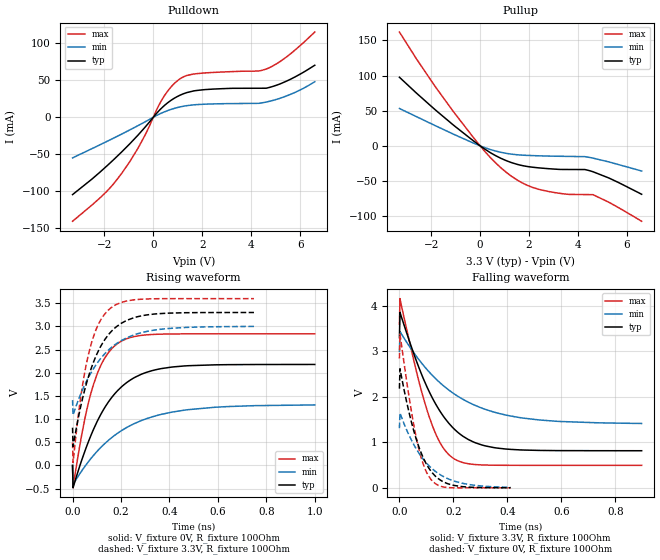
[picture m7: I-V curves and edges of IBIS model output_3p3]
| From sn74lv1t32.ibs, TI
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|   output_3p3 Model
[Model]   output_3p3
Model_type   Output
Polarity   Inverting
Vmeas = 1.65
Vref = 0
Cref = 30pF
Rref = 150
|   typ   min   max
|   (nom PVT)   (fast PVT)   (slow PVT)
C_comp   1.702e-12   1.593e-12   1.765e-12
| Where nom  PVT is Nominal Process, 3.3V, 40C
|   Fast PVT is Strong Process,  3.6V, -40C
|   Slow PVT is Weak Process,   3V, 140C
[Voltage Range]   3.3   3   3.6
|Junction Temperature
[Temperature Range]   40   140   -40
[Pullup Reference]   3.3   3   3.6
[Pulldown Reference]   0   0   0
[Power Clamp Reference]   3.3   3   3.6
[GND Clamp Reference]   0   0   0
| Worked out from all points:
|   slope of the pulldown table from 0 to 0.495 V, typ, clamps not added: 29 ohm
|   slope of the pullup table from 0 to 0.495 V, typ, clamps not added: 43.9 ohm
|   falling waveform, V_fixture 3.3V, R_fixture 100Ohm: 20-80 % time 138ps typ, 225ps min, 93.8ps max; typ from 3.3 V to 0.815 V
|   rising waveform, V_fixture 0V, R_fixture 100Ohm: 20-80 % time 153ps typ, 232ps min, 93.4ps max; typ from 0 V to 2.18 V
|   rising waveform, V_fixture 3.3V, R_fixture 100Ohm: 20-80 % time 110ps typ, 148ps min, 76.2ps max; typ from 0.815 V to 3.3 V
|   falling waveform, V_fixture 0V, R_fixture 100Ohm: 20-80 % time 76.3ps typ, 112ps min, 57ps max; typ from 2.18 V to 0.002 V
[Pulldown]
|   Voltage   I(typ)   I(min)   I(max)
-3.3V     -104.5mA   -54.85mA   -140.5mA
-1.896V   -65.69mA   -32.59mA   -99.89mA
-1.291V   -46.79mA   -22.65mA   -75.76mA
-618mV    -23.85mA   -11.17mA   -41.41mA
408mV     14.56mA    6.683mA    26.68mA
746.4mV   23.38mA    10.87mA    41.78mA
1.049V    29.16mA    13.66mA    51mA
1.373V    33.38mA    15.72mA    56.48mA
2.043V    37.19mA    17.6mA     59.75mA
4.609V    39.26mA    20.53mA    65.09mA
5.448V    48.87mA    28.84mA    81.62mA
6.6V      70.29mA    47.98mA    115.2mA
[Pullup]
|   Voltage   I(typ)   I(min)   I(max)
-3.3V     97.54mA    53.13mA    161.8mA
-1.882V   52.63mA    29.49mA    86.56mA
-1.043V   28.1mA     15.84mA    46.36mA
194.7mV   -4.752mA   -2.606mA   -8.053mA
1.079V    -21.23mA   -10.73mA   -37.97mA
1.736V    -28.14mA   -13.22mA   -52.95mA
2.376V    -31.23mA   -14.13mA   -61.59mA
3.627V    -33.6mA    -15mA      -69.02mA
4.446V    -35.06mA   -16.32mA   -69.31mA
4.61V     -36.79mA   -17.43mA   -69.37mA
5.25V     -45.55mA   -22.74mA   -80.01mA
6.6V      -68.82mA   -35.76mA   -107.2mA
[Ramp]
R_load = 100
|   typ   min   max
dV/dt_r   1.30758/1.52632e-10   0.783735/2.32218e-10   1.70409/9.33057e-11
dV/dt_f   1.49085/1.37591e-10   0.951762/2.2497e-10   1.8634/9.37035e-11
[Falling Waveform]
V_fixture = 3.3V
V_fixture_min = 3V
V_fixture_max = 3.6V
R_fixture = 100Ohm
|   Time   V(typ)   V(min)   V(max)
0s        3.3V       3V         3.6V
2ps       3.858V     3.435V     4.159V
68ps      2.708V     2.849V     2.437V
112ps     2.093V     2.535V     1.535V
152ps     1.669V     2.301V     976.8mV
202ps     1.298V     2.068V     640.4mV
276ps     1.003V     1.824V     514.1mV
366ps     870.9mV    1.64V      496.1mV
580ps     818.3mV    1.463V     494.3mV
898ps     815.2mV    1.414V     494.3mV
[Rising Waveform]
V_fixture = 0V
V_fixture_min = 0V
V_fixture_max = 0V
R_fixture = 100Ohm
|   Time   V(typ)   V(min)   V(max)
0s        426.8pV    5.751nV    702.7pV
2ps       -481.1mV   -412mV     -482.8mV
52ps      324.7mV    -12.69mV   1.04V
76ps      649mV      150.7mV    1.563V
102ps     953.1mV    308.3mV    1.98V
146ps     1.355V     532.6mV    2.42V
202ps     1.696V     751.4mV    2.683V
288ps     1.976V     976.5mV    2.809V
410ps     2.123V     1.15V      2.837V
1ns       2.179V     1.306V     2.84V
[Rising Waveform]
V_fixture = 3.3V
V_fixture_min = 3V
V_fixture_max = 3.6V
R_fixture = 100Ohm
|   Time   V(typ)   V(min)   V(max)
0s        815.2mV    1.411V     494.3mV
2ps       409.2mV    1.087V     60.5mV
22ps      980.7mV    1.386V     1.004V
40ps      1.418V     1.619V     1.692V
80ps      2.139V     2.034V     2.677V
116ps     2.567V     2.307V     3.137V
160ps     2.892V     2.544V     3.406V
222ps     3.126V     2.751V     3.547V
308ps     3.249V     2.893V     3.593V
749ps     3.3V       3V         3.6V
[Falling Waveform]
V_fixture = 0V
V_fixture_min = 0V
V_fixture_max = 0V
R_fixture = 100Ohm
|   Time   V(typ)   V(min)   V(max)
0s        2.179V     1.311V     2.841V
2ps       2.617V     1.645V     3.379V
38ps      1.599V     1.127V     1.912V
66ps      1.004V     820.2mV    1.006V
92ps      613.4mV    601.9mV    461mV
120ps     343.1mV    426.3mV    162mV
156ps     153.9mV    270.6mV    29.05mV
200ps     55.98mV    153.7mV    426.3uV
270ps     12.04mV    62.16mV    617uV
412ps     1.538mV    9.966mV    148.9uV
